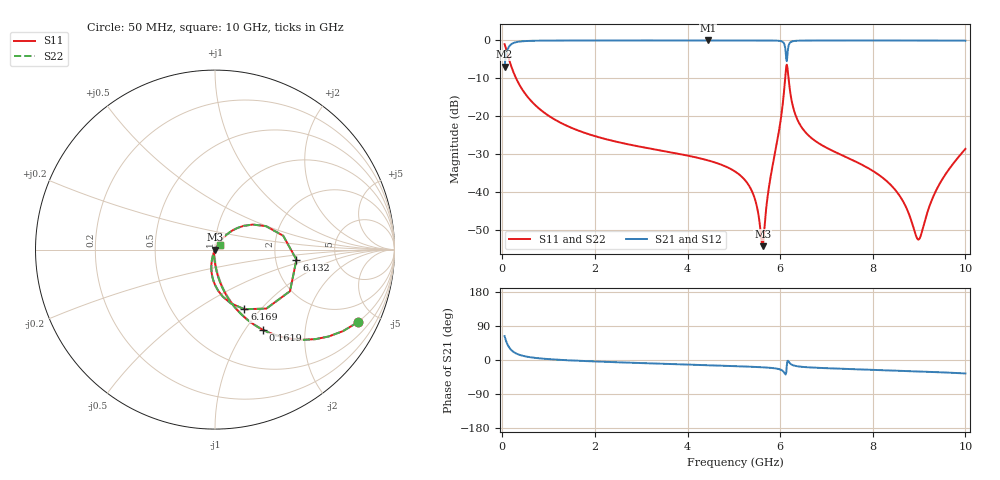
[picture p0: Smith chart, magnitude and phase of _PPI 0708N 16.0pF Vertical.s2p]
! S-Parameter data specifications (vertical orientation):
! Substrate: 40-mil Rogers 3003C, Substrate thickness, H=1.016mm, Dielectric constant, Er=3, Conductor thickness, T_mtl=0.043mm, Loss Tangent, Tand=0.003
! PCB Mounting Pad Footprint: Pad width, PadW=2.54mm , Pad length, PadL=0.51mm , Pad gap, PadG (edge-to-edge)=0.71mm , Reference planes=1.73mm apart
! Created Tue Jan 16 08:52:16 2018
# GHz S MA R 50
! 2 Port Network Data from SP1.SP block
! freq  magS11  angS11  magS21  angS21  magS12  angS12  magS22  angS22
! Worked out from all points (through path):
!   801 points, 50 MHz to 10 GHz, reference 50 ohm
!   highest |S21| = -0.01 dB at 4.44 GHz (marker M1); lowest = -6.9 dB at 50 MHz (marker M2)
!   group delay of S21, straight-line fit = 12.4 ps
!   lowest |S11| = -54.4 dB at 5.622 GHz (marker M3), VSWR 1.00, Z = 50.2 - j0.0528 ohm
!   |S11| at or under -10 dB: 297.4 MHz to 6.108 GHz (5.81 GHz wide, 181 % of centre); 6.181 GHz to end of sweep
!   |S22| runs from -54.4 to -1.0 dB; largest |S21 - S12| = 0
!   S11 on the Smith chart (normalised r, x): 50 MHz: 0.99, -3.93; 161.9 MHz: 0.99, -1.21; 6.132 GHz: 2.62, -0.37; 6.169 GHz: 1.07, -0.82; 10 GHz: 1.05, +0.05
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0.05  0.8924 -27.0  0.4511 63.0  0.4511 63.0  0.8924 -27.0
0.1619375  0.5214 -59.1  0.8531 30.9  0.8531 30.9  0.5214 -59.1
0.323625  0.293 -74.0  0.9559 15.9  0.9559 15.9  0.293 -74.0
0.69675  0.1424 -84.1  0.9895 5.8  0.9895 5.8  0.1424 -84.1
1.716625  0.06193 -92.0  0.9975 -2.4  0.9975 -2.4  0.06193 -92.0
3.370812  0.03553 -98.5  0.9985 -9.6  0.9985 -9.6  0.03553 -98.5
4.440437  0.02599 -101.9  0.9986 -13.8  0.9986 -13.8  0.02599 -101.9
5.025  0.01854 -102.9  0.9986 -16.2  0.9986 -16.2  0.01854 -102.9
5.398125  0.00995 -100.0  0.9983 -17.9  0.9983 -17.9  0.00995 -100.0
5.622  0.001911 -16.0  0.9979 -19.2  0.9979 -19.2  0.001911 -16.0
5.97025  0.0614 57.0  0.9881 -23.9  0.9881 -23.9  0.0614 57.0
6.06975  0.1731 44.0  0.9391 -30.3  0.9391 -30.3  0.1731 44.0
6.131938  0.4572 -7.0  0.5667 -32.1  0.5667 -32.1  0.4572 -7.0
6.16925  0.3705 -63.7  0.7694 -2.0  0.7694 -2.0  0.3705 -63.7
6.231438  0.1819 -91.8  0.9548 -10.9  0.9548 -10.9  0.1819 -91.8
6.343375  0.09887 -102.1  0.9881 -16.0  0.9881 -16.0  0.09887 -102.1
6.691625  0.05036 -107.9  0.9967 -19.9  0.9967 -19.9  0.05036 -107.9
8.345812  0.01306 -110.1  0.9979 -27.4  0.9979 -27.4  0.01306 -110.1
8.65675  0.00742 -103.8  0.9977 -28.7  0.9977 -28.7  0.00742 -103.8
8.992563  0.002342 -29.9  0.9973 -30.2  0.9973 -30.2  0.002342 -29.9
9.403  0.01147 41.3  0.9963 -32.1  0.9963 -32.1  0.01147 41.3
10  0.03685 43.3  0.9917 -35.4  0.9917 -35.4  0.03685 43.3
